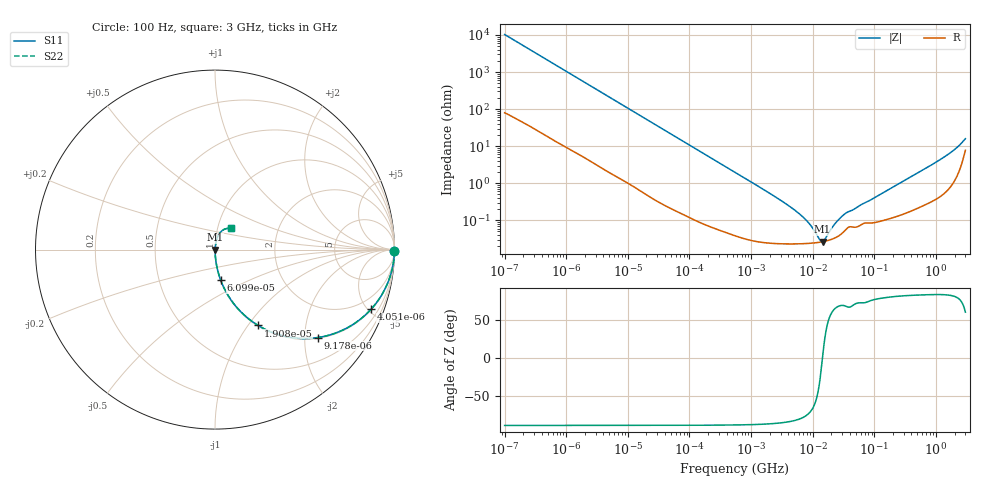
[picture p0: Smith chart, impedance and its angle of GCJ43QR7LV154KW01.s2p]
!Murata Part Number: GCJ43QR7LV154KW01
!These Parameters are Measured in Series Mode Connection
!Data Generated on Mar 13, 2026
!  o--ll--o
!Port1  Port2
!  o------o
!Operation Temp=25[degC], DC Bias Voltage=0[V]
!Freq. Start=100[Hz] Stop=3[GHz] 401[Steps]
# Hz S RI R 50
!Freq.(Hz) S11(Real) S11(Imag) S21(Real) S21(Imag) S12(Real) S12(Imag) S22(Real) S22(Imag)
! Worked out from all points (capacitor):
!   401 points, 100 Hz to 3 GHz, reference 50 ohm
!   read as one part in series: C = 154 nF near 109 Hz
!   lowest |Z| = 26.4 mohm at 14.43 MHz (marker M1)
!   series resonance near 14.38 MHz, so ESL is about 800 pH
!   S11 on the Smith chart (normalised r, x): 100 Hz: open; 4.051 kHz: 1.05, -5.21; 9.178 kHz: 1.02, -2.31; 19.08 kHz: 1.01, -1.12; 60.99 kHz: 1.00, -0.35; 3 GHz: 1.16, +0.28
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100  0.9998 -0.00967  0.000168 0.00967  0.000168 0.00967  0.9998 -0.00967
584  0.9964 -0.0557  0.0036 0.0557  0.0036 0.0557  0.9964 -0.0557
1788  0.9704 -0.1648  0.0296 0.1648  0.0296 0.1648  0.9704 -0.1648
4051  0.8695 -0.3323  0.1305 0.3323  0.1305 0.3323  0.8695 -0.3323
9178  0.5714 -0.4902  0.4286 0.4902  0.4286 0.4902  0.5714 -0.4902
19078  0.24 -0.4225  0.76 0.4225  0.76 0.4225  0.24 -0.4225
31977  0.1027 -0.299  0.8973 0.299  0.8973 0.299  0.1027 -0.299
60986  0.0316 -0.17  0.9684 0.17  0.9684 0.17  0.0316 -0.17
157206  0.0055 -0.0681  0.9945 0.0681  0.9945 0.0681  0.0055 -0.0681
547723  0.000775 -0.0198  0.9992 0.0198  0.9992 0.0198  0.000775 -0.0198
4323298  0.000236 -0.0023  0.9998 0.0023  0.9998 0.0023  0.000236 -0.0023
6941223  0.000235 -0.00121  0.9998 0.00121  0.9998 0.00121  0.000235 -0.00121
9794414  0.000243 -0.000598  0.9998 0.000598  0.9998 0.000598  0.000243 -0.000598
1.268047e7  0.000255 -0.000191  0.9997 0.000191  0.9997 0.000191  0.000255 -0.000191
1.442825e7  0.000264 5.2e-06  0.9997 -5.2e-06  0.9997 -5.2e-06  0.000264 5.2e-06
1.572531e7  0.000272 0.000136  0.9997 -0.000136  0.9997 -0.000136  0.000272 0.000136
2.316512e7  0.000337 0.000753  0.9997 -0.000753  0.9997 -0.000753  0.000337 0.000753
3.268714e7  0.000516 0.00137  0.9995 -0.00137  0.9995 -0.00137  0.000516 0.00137
1.751444e8  0.00115 0.0068  0.9989 -0.0068  0.9989 -0.0068  0.00115 0.0068
1.214989e9  0.00654 0.0446  0.9935 -0.0446  0.9935 -0.0446  0.00654 0.0446
2.219584e9  0.0241 0.0889  0.9759 -0.0889  0.9759 -0.0889  0.0241 0.0889
3e9  0.0872 0.118  0.9128 -0.118  0.9128 -0.118  0.0872 0.118
